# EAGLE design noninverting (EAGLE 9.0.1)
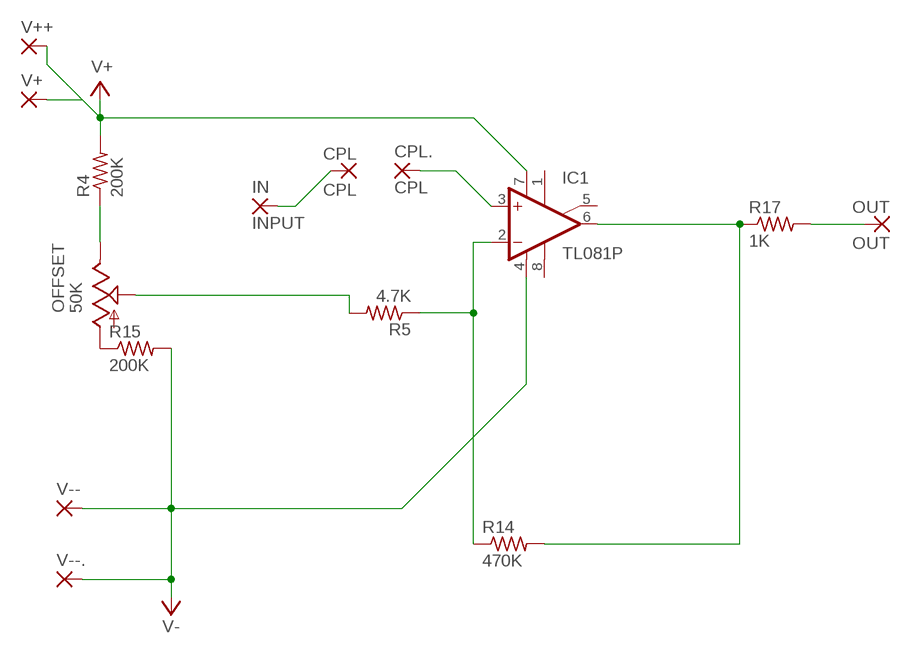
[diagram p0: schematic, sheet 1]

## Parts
CPL  CPL  3,17/1,3  [3,17/1,3]
CPL.  CPL  3,17/1,3  [3,17/1,3]
IC1  TL081P  [DIL08]
IN  INPUT  3,17/1,3  [3,17/1,3]
OFFSET  50K  TRIM_US-S63X  [S63X]
OUT  OUT  3,17/1,3  [3,17/1,3]
R4  200K  R-US_0204/7  [0204/7]
R5  4.7K  R-US_0204/7  [0204/7]
R14  470K  R-US_0204/7  [0204/7]
R15  200K  R-US_0204/7  [0204/7]
R17  1K  R-US_0204/7  [0204/7]
V+  3,17/1,3  [3,17/1,3]
V++  3,17/1,3  [3,17/1,3]
V--  3,17/1,3  [3,17/1,3]
V--.  3,17/1,3  [3,17/1,3]

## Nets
N$1: CPL.1(P) IN.1(P)
N$2: CPL..1(P) IC1.3(+IN)
N$18: IC1.6(OUT) R14.2 R17.1
N$19: OUT.1(P) R17.2
N$20: IC1.2(-IN) R5.1 R14.1
N$22: OFFSET.S R5.2
N$26: OFFSET.A R15.1
N$27: OFFSET.E R4.1
V+: IC1.7(V+) R4.2 V++.1(P) V+.1(P)
V-: IC1.4(V-) R15.2 V--.1(P) V--..1(P)
Unconnected: IC1.1(ON1) IC1.5(ON2) IC1.8(OPT)

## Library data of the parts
CPL CPL. IN OUT V+ V++ V-- V--. = wirepad:3,17/1,3: THROUGH-HOLE PAD
IC1 = linear:TL081: OP AMP
OFFSET = pot:TRIM_US-: POTENTIOMETER
R4 R5 R14 R15 R17 = rcl:R-US_: RESISTOR, American symbol

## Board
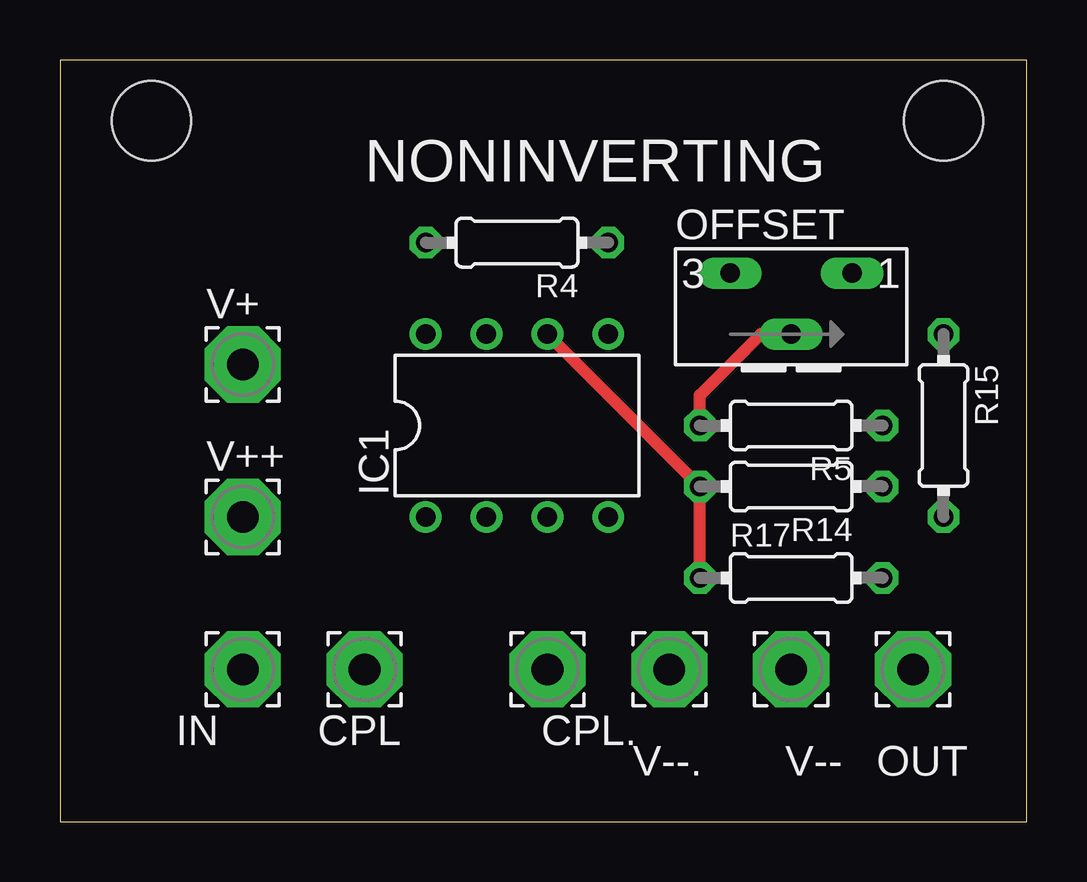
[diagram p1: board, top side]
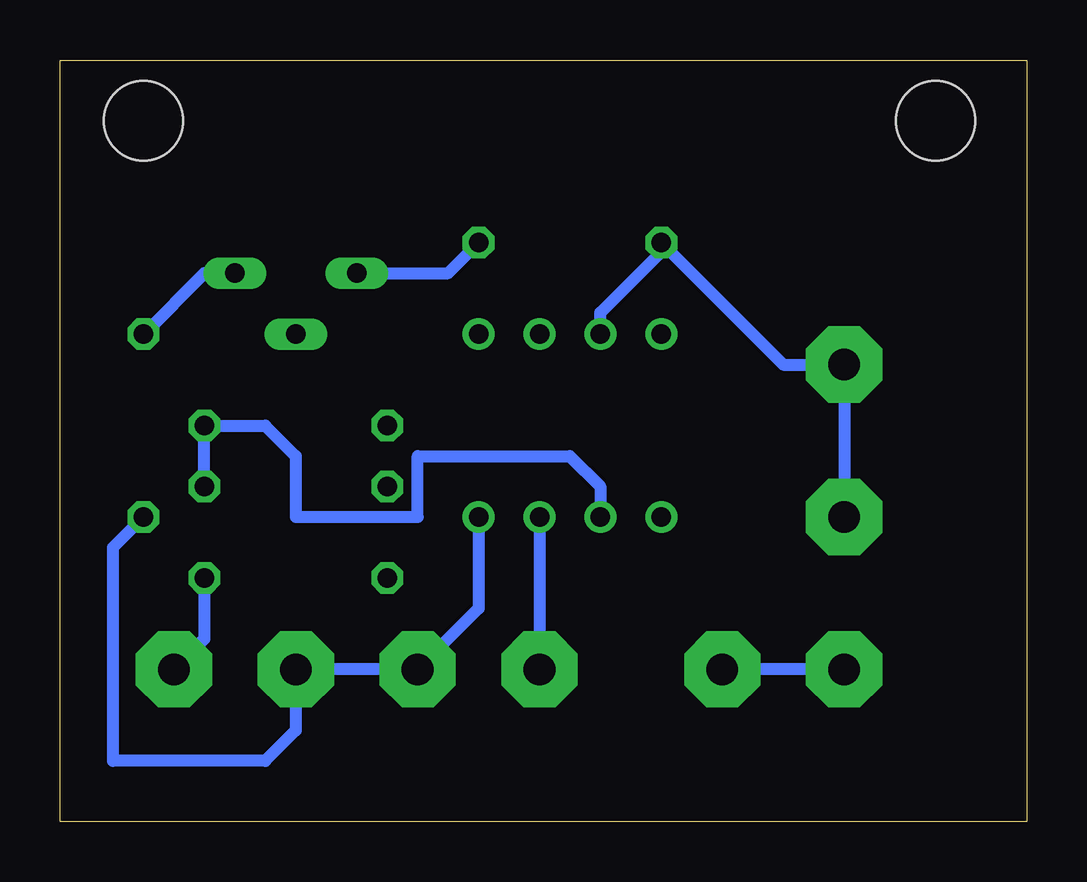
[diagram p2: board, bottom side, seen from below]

Size 40.31 x 31.74 mm. Coordinates in mm from the lower left corner, seen from the top.
Outline: 0,0 40.31,0 40.31,31.74 0,31.74 0,0
Copper layers (1*16): Top 0.035mm / dielectric 1.5mm / Bottom 0.035mm
Design rules "default": minimum track width 6mil, minimum drill 0.35mm, track to track 6mil, track to pad 6mil, pad to pad 6mil, via to via 6mil, smd to smd 6mil, copper to edge 40mil, drill to drill 6mil, minimum pad ring 10mil, minimum via ring 8mil, stop-mask expansion 4mil, vias tented up to drill 0mil, thermal gap 10mil
Holes 3.3 mm at 3.81,29.21 36.83,29.21

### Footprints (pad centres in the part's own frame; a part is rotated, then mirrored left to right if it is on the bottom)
3,17/1,3 = drill 1.321 pad 3.175 octagon: 1 0,0
DIL08 = drill 0.813 pad 1.27: 1 -3.81,-3.81; 2 -1.27,-3.81; 3 1.27,-3.81; 4 3.81,-3.81; 5 3.81,3.81; 6 1.27,3.81; 7 -1.27,3.81; 8 -3.81,3.81
S63X = drill 0.813 long: A 2.54,0; E -2.54,0; S 0,-2.54
0204/7 = drill 0.813 octagon: 1 -3.81,0; 2 3.81,0

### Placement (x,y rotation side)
CPL  12.7,6.35 180 top
CPL.  20.32,6.35 0 top
IC1  19.05,16.51 0 top
IN  7.62,6.35 0 top
OFFSET  30.48,22.86 0 top
OUT  35.56,6.35 0 top
R4  19.05,24.13 180 top
R5  30.48,16.51 180 top
R14  30.48,13.97 180 top
R15  36.83,16.51 270 top
R17  30.48,10.16 0 top
V+  7.62,19.05 0 top
V++  7.62,12.7 0 top
V--  30.48,6.35 0 top
V--.  25.4,6.35 0 top

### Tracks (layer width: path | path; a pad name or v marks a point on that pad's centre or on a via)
N$1
  Bottom 0.508: IN.1 CPL.1
N$2
  Bottom 0.508: IC1.3 CPL..1
N$18
  Top 0.508: 26.64,14 R14.2 | 26.64,14 IC1.6 | R17.1 R14.2 | R14.2 26.64,14
N$19
  Bottom 0.508: R17.2 34.29,7.62 OUT.1
N$20
  Bottom 0.508: R14.1 R5.1 31.75,16.51 30.48,15.24 30.48,12.7 25.4,12.7 25.4,15.24 19.05,15.24 17.78,13.97 IC1.2
N$22
  Top 0.508: R5.2 26.67,17.78 29.21,20.32 OFFSET.S
N$26
  Bottom 0.508: OFFSET.A 34.29,22.86 R15.1
N$27
  Bottom 0.508: OFFSET.E 24.13,22.86 R4.1
V+
  Bottom 0.508: 15.05,23.94 10.16,19.05 V+.1 V++.1 | 15.05,23.94 R4.2 | IC1.7 17.78,21.22 15.05,23.94
V-
  Bottom 0.508: IC1.4 22.86,8.89 V--..1 V--.1 30.48,3.81 31.75,2.54 38.1,2.54 38.1,11.43 R15.2

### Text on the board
tNames: NONINVERTING
tValues: MICROGAIN!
